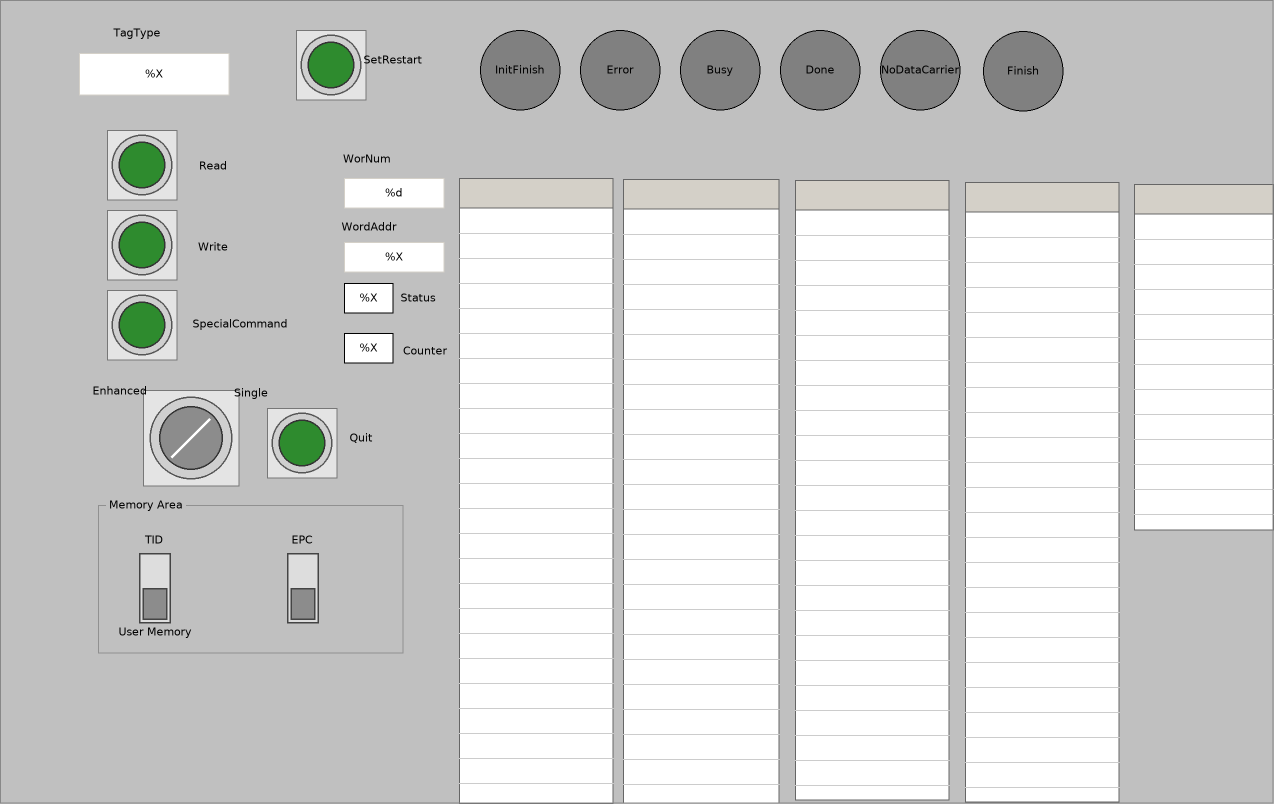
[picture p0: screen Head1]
VISUALIZATION Head1  // 1274x804
    GroupBox (98,497 305x156), "Memory Area"
        DipSwitch (22,56 70x70), variable: MAIN.Head1UserMemoryUID, behaviour: TOGGLE, style: Switch-DipSwitch-Gray
        DipSwitch (170,56 70x70), variable: MAIN.Head1EPC, behaviour: TOGGLE, style: Switch-DipSwitch-Gray
        Label (129,28 150x30), "EPC"
    PushSwitch (107,130 70x70), variable: MAIN.Head1Read, behaviour: TAP, style: Switch-PushSwitch-Green
    PushSwitch (107,210 70x70), variable: MAIN.Head1Write, behaviour: TAP, style: Switch-PushSwitch-Green
    RotarySwitch (138,390 106x96), variable: MAIN.Head1SingleEnhanced, behaviour: TOGGLE, style: Switch-RotarySwitch-Gray
    Textfield (79,53 150x42), "%X", tooltip "TagType", text variable: MAIN.Head1TagType
        OnMouseDown: write MAIN.Head1TagType via Default
    Table (459,178 154x626), data array: MAIN.IDENTControl_FB_Head1.INDATA
        p1892666644: MAIN.Data_Channel.InData[2][INDEX]
        p3854506369: MAIN.IDENTControl_FB_Head1.INDATA[INDEX]
    Table (623,179 156x624), data array: MAIN.IDENTControl_FB_Head1.OUTDATA
        p1892666644: MAIN.Data_Channel.OutData[2][INDEX]
        p3854506369: MAIN.IDENTControl_FB_Head1.OUTDATA[INDEX]
        Columns.Column.[0].Template: OnMouseDown: write the text variable via Default
    Textfield (344,242 100x30), "%X", text variable: MAIN.Head1StartAddress
        OnMouseClick: write MAIN.Head1StartAddress via Default
    Textfield (344,178 100x30), "%d", text variable: MAIN.Head1WordNum
        OnMouseClick: write MAIN.Head1WordNum via Default
    PushSwitch (296,30 70x70), variable: MAIN.Head1SetRestart, behaviour: TAP, style: Switch-PushSwitch-Green
    PushSwitch (267,408 70x70), tooltip "Cancel "Enhanced"-Command", variable: MAIN.Head1Quit, behaviour: TAP, style: Switch-PushSwitch-Green
    PushSwitch (107,290 70x70), variable: MAIN.Head1SpecialCommand, behaviour: TAP, style: Switch-PushSwitch-Green
    Table (1134,184 140x346), data array: MAIN.IDENTControl_FB_Head1.UserData.SpecialCommand
        p1892666644: MAIN.Data_Channel.SpecialCommand[2][INDEX]
        p3854506369: MAIN.IDENTControl_FB_Head1.UserData.SpecialCommand[INDEX]
        Columns.Column.[0].Template: OnMouseDown: write the text variable via Default
    Rectangle (344,283 49x30), "%X", text variable: MAIN.Head1Status, input disabled if: TRUE
    Rectangle (344,333 49x30), "%X", text variable: MAIN.Head1ReplyCounter, input disabled if: TRUE
    Ellipse (480,30 80x80), "InitFinish", colour toggle: MAIN.Head1InitFinish
    Ellipse (580,30 80x80), "Error", colour toggle: MAIN.Head1Error
    Ellipse (680,30 80x80), "Busy", colour toggle: MAIN.Head1Busy
    Ellipse (780,30 80x80), "Done", colour toggle: MAIN.Head1Done
    Ellipse (880,30 80x80), "NoDataCarrier", colour toggle: MAIN.Head1NoDataCarrier
    Label (62,18 150x30), "TagType"
    Label (292,144 150x30), "WorNum"
    Label (294,212 150x30), "WordAddr"
    Label (343,283 150x30), "Status"
    Label (350,336 150x30), "Counter"
    Label (138,151 150x30), "Read"
    Label (138,232 150x30), "Write"
    Label (165,309 150x30), "SpecialCommand"
    Label (45,376 150x30), "Enhanced"
    Label (176,378 150x30), "Single"
    Label (286,423 150x30), "Quit"
    Label (79,525 150x30), "TID"
    Label (80,617 150x30), "User Memory"
    Ellipse (983,31 80x80), "Finish", colour toggle: MAIN.Head1Finish
    Table (795,180 154x620), data array: MAIN.IDENTControl_FB_Head1.UserData.ReadData
        p1892666644: MAIN.Data_Channel.SpecialCommand[2][INDEX]
        p3854506369: MAIN.IDENTControl_FB_Head1.UserData.ReadData[INDEX]
        Columns.Column.[0].Template: OnMouseDown: write the text variable via Default
    Table (965,182 154x620), data array: MAIN.IDENTControl_FB_Head1.UserData.WriteData
        p1892666644: MAIN.Data_Channel.SpecialCommand[2][INDEX]
        p3854506369: MAIN.IDENTControl_FB_Head1.UserData.WriteData[INDEX]
        Columns.Column.[0].Template: OnMouseDown: write the text variable via Default
    Label (318,45 150x30), "SetRestart"
END_VISUALIZATION
